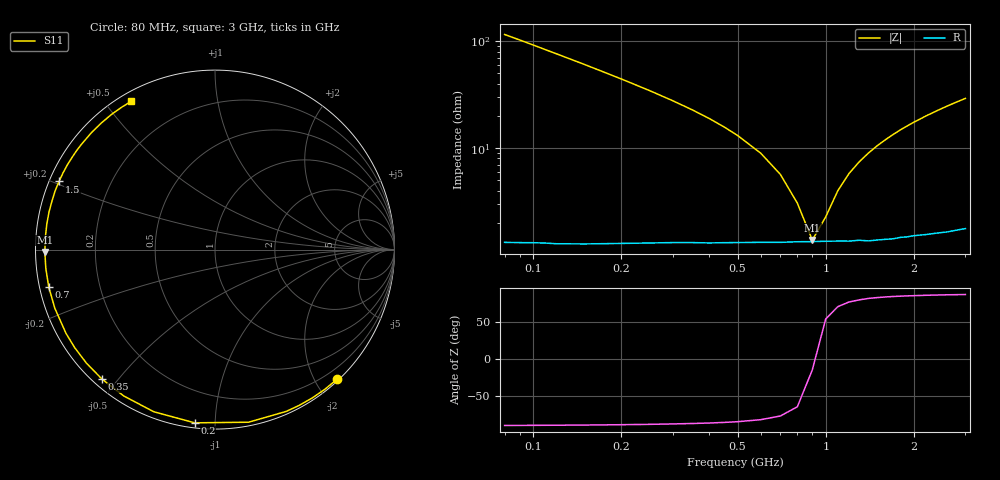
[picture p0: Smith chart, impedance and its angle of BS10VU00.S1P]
! SIEMENS Small Signal Semiconductors
! BB640
! Si Tuning Diode in SOD323
! VR = 10 V
! S-Parameters:  July  1993
# GHz  S  MA  R  50
!  f  S11
! GHz  MAG  ANG
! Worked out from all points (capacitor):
!   33 points, 80 MHz to 3 GHz, reference 50 ohm
!   read as one part to ground: C = 17 pF near 80 MHz
!   lowest |Z| = 1.38 ohm at 900 MHz (marker M1)
!   series resonance near 916 MHz, so ESL is about 1.8 nH
!   S11 on the Smith chart (normalised r, x): 80 MHz: 0.03, -2.32; 200 MHz: 0.03, -0.89; 350 MHz: 0.03, -0.46; 700 MHz: 0.03, -0.11; 1.5 GHz: 0.03, +0.21; 3 GHz: 0.04, +0.58
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0.08  0.9918 -46.7
0.1  0.9883 -56.8
0.11  0.9865 -61.7
0.12  0.9849 -66.3
0.15  0.9797 -79.0
0.2  0.9718 -96.7
0.25  0.9656 -110.7
0.3  0.9609 -121.9
0.35  0.9577 -131.0
0.4  0.9557 -138.6
0.45  0.9537 -145.1
0.5  0.9523 -150.7
0.6  0.9504 -159.9
0.7  0.9495 -167.4
0.8  0.9484 -173.7
0.9  0.9481 -179.2
1  0.9478 175.8
1.2  0.9482 167.2
1.4  0.9489 159.8
1.5  0.9485 156.4
1.6  0.9484 153.2
1.8  0.9477 147.1
2  0.9474 141.6
2.2  0.9479 136.5
2.4  0.948 131.8
2.6  0.9486 127.4
2.8  0.9485 123.3
3  0.9487 119.5
